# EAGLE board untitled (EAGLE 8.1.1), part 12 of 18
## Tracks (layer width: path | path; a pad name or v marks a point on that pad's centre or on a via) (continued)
S$11975 (continued)
  Bottom 0: 16.56,150.84 16.82,151.06
S$11976
  Bottom 0: 16.82,151.06 17.03,151.35
S$11977
  Bottom 0: 17.03,151.35 17.16,151.67
S$11978
  Bottom 0: 17.16,151.67 17.21,152.02
S$11979
  Bottom 0: 17.21,152.02 17.16,152.36
S$11980
  Bottom 0: 17.16,152.36 17.03,152.69
S$11981
  Bottom 0: 17.03,152.69 16.82,152.97
S$11982
  Bottom 0: 16.82,152.97 16.56,153.2
S$11983
  Bottom 0: 16.56,153.2 16.24,153.35
S$11984
  Bottom 0: 16.24,153.35 15.89,153.41
S$11985
  Bottom 0: 15.89,153.41 15.54,153.39
S$11986
  Bottom 0: 15.54,153.39 15.24,153.29
S$11987
  Bottom 0: 15.24,153.29 16.21,154.26
S$11988
  Bottom 0: 16.21,154.26 16.27,154.33
S$11989
  Bottom 0: 16.27,154.33 16.32,154.41
S$11990
  Bottom 0: 16.32,154.41 16.36,154.49
S$11991
  Bottom 0: 16.36,154.49 16.38,154.57
S$11992
  Bottom 0: 16.38,154.57 16.38,154.66
S$11993
  Bottom 0: 16.38,154.66 16.38,161.85
S$11994
  Bottom 0: 16.38,161.85 16.62,162.02
S$11995
  Bottom 0: 16.62,162.02 16.83,162.28
S$11996
  Bottom 0: 16.83,162.28 16.96,162.57
S$11997
  Bottom 0: 16.96,162.57 17,162.89
S$11998
  Bottom 0: 17,162.89 16.96,163.22
S$11999
  Bottom 0: 16.96,163.22 16.83,163.51
S$12000
  Bottom 0: 16.83,163.51 16.62,163.77
S$12001
  Bottom 0: 16.62,163.77 16.36,163.96
S$12002
  Bottom 0: 16.36,163.96 16.06,164.06
S$12003
  Bottom 0: 16.06,164.06 15.73,164.08
S$12004
  Bottom 0: 15.73,164.08 15.41,164.02
S$12005
  Bottom 0: 15.41,164.02 15.12,163.87
S$12006
  Bottom 0: 15.12,163.87 14.89,163.65
S$12007
  Bottom 0: 14.89,163.65 14.77,163.46
S$12008
  Bottom 0: 14.77,163.46 13.65,163.46
S$12009
  Bottom 0: 13.65,163.46 12.19,164.93
S$12010
  Bottom 0: 12.19,164.93 12.2,164.95
S$12011
  Bottom 0: 12.2,164.95 12.24,165.27
S$12012
  Bottom 0: 12.24,165.27 12.2,165.59
S$12013
  Bottom 0: 12.2,165.59 12.07,165.89
S$12014
  Bottom 0: 12.07,165.89 11.86,166.14
S$12015
  Bottom 0: 11.86,166.14 11.6,166.33
S$12016
  Bottom 0: 11.6,166.33 11.29,166.44
S$12017
  Bottom 0: 11.29,166.44 10.97,166.46
S$12018
  Bottom 0: 10.97,166.46 10.65,166.39
S$12019
  Bottom 0: 10.65,166.39 10.36,166.24
S$12020
  Bottom 0: 10.36,166.24 10.12,166.02
S$12021
  Bottom 0: 10.12,166.02 9.97,165.79
S$12022
  Bottom 0: 9.97,165.79 9.97,170.19
S$12023
  Bottom 0: 9.97,170.19 10.16,169.99
S$12024
  Bottom 0: 10.16,169.99 10.46,169.8
S$12025
  Bottom 0: 10.46,169.8 10.78,169.7
S$12026
  Bottom 0: 10.78,169.7 11.13,169.68
S$12027
  Bottom 0: 11.13,169.68 11.48,169.74
S$12028
  Bottom 0: 11.48,169.74 11.66,169.82
S$12029
  Bottom 0: 11.66,169.82 22,159.49
S$12030
  Bottom 0: 22,159.49 21.9,159.55
S$12031
  Bottom 0: 21.9,159.55 21.61,159.61
S$12032
  Bottom 0: 21.61,159.61 21.3,159.59
S$12033
  Bottom 0: 21.3,159.59 21.02,159.48
S$12034
  Bottom 0: 21.02,159.48 20.78,159.29
S$12035
  Bottom 0: 20.78,159.29 20.61,159.04
S$12036
  Bottom 0: 20.61,159.04 20.52,158.75
S$12037
  Bottom 0: 20.52,158.75 20.52,158.45
S$12038
  Bottom 0: 20.52,158.45 20.61,158.16
S$12039
  Bottom 0: 20.61,158.16 20.78,157.91
S$12040
  Bottom 0: 20.78,157.91 21.02,157.72
S$12041
  Bottom 0: 21.02,157.72 21.3,157.61
S$12042
  Bottom 0: 21.3,157.61 21.61,157.59
S$12043
  Bottom 0: 21.61,157.59 21.9,157.66
S$12044
  Bottom 0: 21.9,157.66 22.16,157.81
S$12045
  Bottom 0: 22.16,157.81 22.29,157.95
S$12046
  Bottom 0: 22.29,157.95 22.29,151.64
S$12047
  Bottom 0: 22.29,151.64 22.16,151.78
S$12048
  Bottom 0: 22.16,151.78 21.9,151.93
S$12049
  Bottom 0: 21.9,151.93 21.61,151.99
S$12050
  Bottom 0: 21.61,151.99 21.3,151.97
S$12051
  Bottom 0: 21.3,151.97 21.02,151.86
S$12052
  Bottom 0: 21.02,151.86 20.78,151.67
S$12053
  Bottom 0: 20.78,151.67 20.61,151.43
S$12054
  Bottom 0: 20.61,151.43 20.52,151.13
S$12055
  Bottom 0: 20.52,151.13 20.52,150.83
S$12056
  Bottom 0: 20.52,150.83 20.61,150.54
S$12057
  Bottom 0: 20.61,150.54 20.78,150.29
S$12058
  Bottom 0: 20.78,150.29 21.02,150.1
S$12059
  Bottom 0: 21.02,150.1 21.3,149.99
S$12060
  Bottom 0: 21.3,149.99 21.61,149.97
S$12061
  Bottom 0: 21.61,149.97 21.9,150.04
S$12062
  Bottom 0: 21.9,150.04 22.16,150.19
S$12063
  Bottom 0: 22.16,150.19 22.29,150.33
S$12064
  Bottom 0: 22.29,150.33 22.29,148.03
S$12065
  Bottom 0: 22.29,148.03 20.8,146.55
S$12066
  Bottom 0: 20.8,146.55 20.76,146.5
S$12067
  Bottom 0: 20.76,146.5 20.72,146.44
S$12068
  Bottom 0: 20.72,146.44 20.69,146.38
S$12069
  Bottom 0: 20.69,146.38 20.67,146.31
S$12070
  Bottom 0: 20.67,146.31 20.67,146.24
S$12071
  Bottom 0: 20.67,146.24 20.67,126.54
S$12072
  Bottom 0: 20.67,126.54 18.82,124.69
S$12073
  Bottom 0: 18.82,124.69 18.78,124.64
S$12074
  Bottom 0: 18.78,124.64 18.74,124.58
S$12075
  Bottom 0: 18.74,124.58 18.71,124.52
S$12076
  Bottom 0: 18.71,124.52 18.69,124.45
S$12077
  Bottom 0: 18.69,124.45 18.69,124.38
S$12078
  Bottom 0: 18.69,124.38 18.69,122.68
S$12079
  Bottom 0: 18.69,122.68 16.99,122.68
S$12080
  Bottom 0: 16.99,122.68 16.91,122.67
S$12081
  Bottom 0: 16.91,122.67 16.84,122.63
S$12082
  Bottom 0: 16.84,122.63 16.78,122.58
S$12083
  Bottom 0: 16.78,122.58 16.74,122.5
S$12084
  Bottom 0: 16.74,122.5 16.73,122.43
S$12085
  Bottom 0: 16.73,122.43 16.73,120.65
S$12086
  Bottom 0: 16.73,120.65 16.74,120.57
S$12087
  Bottom 0: 16.74,120.57 16.78,120.5
S$12088
  Bottom 0: 16.78,120.5 16.84,120.45
S$12089
  Bottom 0: 16.84,120.45 16.91,120.41
S$12090
  Bottom 0: 16.91,120.41 16.99,120.4
S$12091
  Bottom 0: 16.99,120.4 18.77,120.4
S$12092
  Bottom 0: 18.77,120.4 18.84,120.41
S$12093
  Bottom 0: 18.84,120.41 18.91,120.45
S$12094
  Bottom 0: 18.91,120.45 18.92,120.45
S$12095
  Bottom 0: 18.92,120.45 22.51,116.85
S$12096
  Bottom 0: 22.51,116.85 22.51,115.23
S$12097
  Bottom 0: 22.51,115.23 22.36,115.18
S$12098
  Bottom 0: 22.36,115.18 22.07,115
S$12099
  Bottom 0: 22.07,115 21.83,114.74
S$12100
  Bottom 0: 21.83,114.74 21.66,114.43
S$12101
  Bottom 0: 21.66,114.43 21.57,114.09
S$12102
  Bottom 0: 21.57,114.09 21.57,113.75
S$12103
  Bottom 0: 21.57,113.75 21.66,113.41
S$12104
  Bottom 0: 21.66,113.41 21.83,113.1
S$12105
  Bottom 0: 21.83,113.1 22.07,112.84
S$12106
  Bottom 0: 22.07,112.84 22.36,112.65
S$12107
  Bottom 0: 22.36,112.65 22.69,112.55
S$12108
  Bottom 0: 22.69,112.55 23.04,112.53
S$12109
  Bottom 0: 23.04,112.53 23.11,112.54
S$12110
  Bottom 0: 23.11,112.54 13.63,103.06
S$12111
  Bottom 0: 13.63,103.06 11.87,103.06
S$12112
  Bottom 0: 16.69,109.99 17.04,110.05
S$12113
  Bottom 0: 17.04,110.05 17.35,110.2
S$12114
  Bottom 0: 17.35,110.2 17.62,110.42
S$12115
  Bottom 0: 17.62,110.42 17.83,110.71
S$12116
  Bottom 0: 17.83,110.71 17.95,111.03
S$12117
  Bottom 0: 17.95,111.03 18,111.38
S$12118
  Bottom 0: 18,111.38 17.95,111.72
S$12119
  Bottom 0: 17.95,111.72 17.83,112.05
S$12120
  Bottom 0: 17.83,112.05 17.62,112.33
S$12121
  Bottom 0: 17.62,112.33 17.35,112.56
S$12122
  Bottom 0: 17.35,112.56 17.04,112.71
S$12123
  Bottom 0: 17.04,112.71 16.69,112.77
S$12124
  Bottom 0: 16.69,112.77 16.34,112.75
S$12125
  Bottom 0: 16.34,112.75 16.01,112.64
S$12126
  Bottom 0: 16.01,112.64 15.72,112.46
S$12127
  Bottom 0: 15.72,112.46 15.48,112.2
S$12128
  Bottom 0: 15.48,112.2 15.3,111.89
S$12129
  Bottom 0: 15.3,111.89 15.22,111.55
S$12130
  Bottom 0: 15.22,111.55 15.22,111.21
S$12131
  Bottom 0: 15.22,111.21 15.3,110.87
S$12132
  Bottom 0: 15.3,110.87 15.48,110.56
S$12133
  Bottom 0: 15.48,110.56 15.72,110.3
S$12134
  Bottom 0: 15.72,110.3 16.01,110.11
S$12135
  Bottom 0: 16.01,110.11 16.34,110.01
S$12136
  Bottom 0: 16.34,110.01 16.69,109.99
S$12137
  Bottom 0: 19.15,114.17 19.59,114.22
S$12138
  Bottom 0: 19.59,114.22 20.02,114.35
S$12139
  Bottom 0: 20.02,114.35 20.42,114.56
S$12140
  Bottom 0: 20.42,114.56 20.76,114.84
S$12141
  Bottom 0: 20.76,114.84 21.05,115.19
S$12142
  Bottom 0: 21.05,115.19 21.26,115.58
S$12143
  Bottom 0: 21.26,115.58 21.38,116.01
S$12144
  Bottom 0: 21.38,116.01 21.43,116.46
S$12145
  Bottom 0: 21.43,116.46 21.38,116.91
S$12146
  Bottom 0: 21.38,116.91 21.26,117.33
S$12147
  Bottom 0: 21.26,117.33 21.05,117.73
S$12148
  Bottom 0: 21.05,117.73 20.76,118.07
S$12149
  Bottom 0: 20.76,118.07 20.42,118.36
S$12150
  Bottom 0: 20.42,118.36 20.02,118.57
S$12151
  Bottom 0: 20.02,118.57 19.59,118.7
S$12152
  Bottom 0: 19.59,118.7 19.15,118.75
S$12153
  Bottom 0: 19.15,118.75 18.7,118.7
S$12154
  Bottom 0: 18.7,118.7 18.27,118.57
S$12155
  Bottom 0: 18.27,118.57 17.88,118.36
S$12156
  Bottom 0: 17.88,118.36 17.53,118.07
S$12157
  Bottom 0: 17.53,118.07 17.24,117.73
S$12158
  Bottom 0: 17.24,117.73 17.03,117.33
S$12159
  Bottom 0: 17.03,117.33 16.91,116.91
S$12160
  Bottom 0: 16.91,116.91 16.86,116.46
S$12161
  Bottom 0: 16.86,116.46 16.91,116.01
S$12162
  Bottom 0: 16.91,116.01 17.03,115.58
S$12163
  Bottom 0: 17.03,115.58 17.24,115.19
S$12164
  Bottom 0: 17.24,115.19 17.53,114.84
S$12165
  Bottom 0: 17.53,114.84 17.88,114.56
S$12166
  Bottom 0: 17.88,114.56 18.27,114.35
S$12167
  Bottom 0: 18.27,114.35 18.7,114.22
S$12168
  Bottom 0: 18.7,114.22 19.15,114.17
S$12169
  Bottom 0: 297.48,103.13 297.48,103.37
S$12170
  Bottom 0: 297.48,103.37 297.47,103.44
S$12171
  Bottom 0: 297.47,103.44 297.43,103.52
S$12172
  Bottom 0: 297.43,103.52 297.37,103.57
S$12173
  Bottom 0: 297.37,103.57 297.3,103.61
S$12174
  Bottom 0: 297.3,103.61 297.23,103.62
S$12175
  Bottom 0: 297.23,103.62 296.15,103.62
S$12176
  Bottom 0: 296.15,103.62 296.15,103.74
S$12177
  Bottom 0: 296.15,103.74 296.13,103.8
S$12178
  Bottom 0: 296.13,103.8 296.13,103.86
S$12179
  Bottom 0: 296.13,103.86 296.1,103.91
S$12180
  Bottom 0: 296.1,103.91 296.09,103.97
S$12181
  Bottom 0: 296.09,103.97 296.05,104
S$12182
  Bottom 0: 296.05,104 296.02,104.05
S$12183
  Bottom 0: 296.02,104.05 294.98,105.1
S$12184
  Bottom 0: 294.98,105.1 295,105.12
S$12185
  Bottom 0: 295,105.12 295.12,105.42
S$12186
  Bottom 0: 295.12,105.42 295.17,105.74
S$12187
  Bottom 0: 295.17,105.74 295.12,106.06
S$12188
  Bottom 0: 295.12,106.06 295,106.36
S$12189
  Bottom 0: 295,106.36 294.79,106.61
S$12190
  Bottom 0: 294.79,106.61 294.52,106.8
S$12191
  Bottom 0: 294.52,106.8 294.22,106.91
S$12192
  Bottom 0: 294.22,106.91 293.89,106.93
S$12193
  Bottom 0: 293.89,106.93 293.57,106.86
S$12194
  Bottom 0: 293.57,106.86 293.47,106.81
S$12195
  Bottom 0: 293.47,106.81 298.16,111.51
S$12196
  Bottom 0: 298.16,111.51 298.2,111.56
S$12197
  Bottom 0: 298.2,111.56 298.24,111.62
S$12198
  Bottom 0: 298.24,111.62 298.27,111.68
S$12199
  Bottom 0: 298.27,111.68 298.28,111.75
S$12200
  Bottom 0: 298.28,111.75 298.29,111.82
S$12201
  Bottom 0: 298.29,111.82 298.29,112.98
S$12202
  Bottom 0: 298.29,112.98 299.41,114.1
S$12203
  Bottom 0: 299.41,114.1 299.4,114.07
S$12204
  Bottom 0: 299.4,114.07 299.4,113.73
S$12205
  Bottom 0: 299.4,113.73 299.49,113.39
S$12206
  Bottom 0: 299.49,113.39 299.66,113.08
S$12207
  Bottom 0: 299.66,113.08 299.82,112.9
S$12208
  Bottom 0: 299.82,112.9 299.82,103.26
S$12209
  Bottom 0: 299.82,103.26 299.76,103.34
S$12210
  Bottom 0: 299.76,103.34 299.48,103.52
S$12211
  Bottom 0: 299.48,103.52 299.17,103.61
S$12212
  Bottom 0: 299.17,103.61 298.85,103.61
S$12213
  Bottom 0: 298.85,103.61 298.53,103.52
S$12214
  Bottom 0: 298.53,103.52 298.44,103.46
S$12215
  Bottom 0: 298.44,103.46 298.32,103.48
S$12216
  Bottom 0: 298.32,103.48 298.02,103.46
S$12217
  Bottom 0: 298.02,103.46 297.74,103.35
S$12218
  Bottom 0: 297.74,103.35 297.5,103.17
S$12219
  Bottom 0: 297.5,103.17 297.48,103.13
S$12220
  Bottom 0: 300.71,106.53 300.71,112.52
S$12221
  Bottom 0: 300.71,112.52 300.87,112.51
S$12222
  Bottom 0: 300.87,112.51 301.18,112.56
S$12223
  Bottom 0: 301.18,112.56 301.29,112.53
S$12224
  Bottom 0: 301.29,112.53 301.63,112.51
S$12225
  Bottom 0: 301.63,112.51 301.98,112.57
S$12226
  Bottom 0: 301.98,112.57 302.3,112.72
S$12227
  Bottom 0: 302.3,112.72 302.56,112.94
S$12228
  Bottom 0: 302.56,112.94 302.63,113.03
S$12229
  Bottom 0: 302.63,113.03 302.63,107.58
S$12230
  Bottom 0: 302.63,107.58 301.93,106.88
S$12231
  Bottom 0: 301.93,106.88 301.84,106.91
S$12232
  Bottom 0: 301.84,106.91 301.51,106.93
S$12233
  Bottom 0: 301.51,106.93 301.19,106.86
S$12234
  Bottom 0: 301.19,106.86 300.9,106.72
S$12235
  Bottom 0: 300.9,106.72 300.71,106.53
S$12236
  Bottom 0: 34.94,107.82 21.52,121.24
S$12237
  Bottom 0: 21.52,121.24 21.56,121.54
S$12238
  Bottom 0: 21.56,121.54 21.51,121.86
S$12239
  Bottom 0: 21.51,121.86 21.38,122.16
S$12240
  Bottom 0: 21.38,122.16 21.16,122.4
S$12241
  Bottom 0: 21.16,122.4 20.89,122.58
S$12242
  Bottom 0: 20.89,122.58 20.58,122.67
S$12243
  Bottom 0: 20.58,122.67 20.25,122.67
S$12244
  Bottom 0: 20.25,122.67 19.94,122.58
S$12245
  Bottom 0: 19.94,122.58 19.67,122.4
S$12246
  Bottom 0: 19.67,122.4 19.57,122.29
S$12247
  Bottom 0: 19.57,122.29 19.57,124.2
S$12248
  Bottom 0: 19.57,124.2 21.42,126.04
S$12249
  Bottom 0: 21.42,126.04 21.47,126.1
S$12250
  Bottom 0: 21.47,126.1 21.5,126.15
S$12251
  Bottom 0: 21.5,126.15 21.53,126.22
S$12252
  Bottom 0: 21.53,126.22 21.55,126.28
S$12253
  Bottom 0: 21.55,126.28 21.55,126.36
S$12254
  Bottom 0: 21.55,126.36 21.55,146.06
S$12255
  Bottom 0: 21.55,146.06 23.04,147.54
S$12256
  Bottom 0: 23.04,147.54 23.09,147.59
S$12257
  Bottom 0: 23.09,147.59 23.12,147.65
S$12258
  Bottom 0: 23.12,147.65 23.16,147.71
S$12259
  Bottom 0: 23.16,147.71 23.17,147.78
S$12260
  Bottom 0: 23.17,147.78 23.18,147.85
S$12261
  Bottom 0: 23.18,147.85 23.18,152.26
S$12262
  Bottom 0: 23.18,152.26 29.48,152.26
S$12263
  Bottom 0: 29.48,152.26 29.58,152.15
S$12264
  Bottom 0: 29.58,152.15 29.8,152.04
S$12265
  Bottom 0: 29.8,152.04 30.05,152.02
S$12266
  Bottom 0: 30.05,152.02 30.3,152.09
S$12267
  Bottom 0: 30.3,152.09 30.39,152.16
S$12268
  Bottom 0: 30.39,152.16 30.47,152.06
S$12269
  Bottom 0: 30.47,152.06 30.67,151.85
S$12270
  Bottom 0: 30.67,151.85 30.72,151.81
S$12271
  Bottom 0: 30.72,151.81 30.78,151.77
S$12272
  Bottom 0: 30.78,151.77 30.85,151.74
S$12273
  Bottom 0: 30.85,151.74 30.91,151.72
S$12274
  Bottom 0: 30.91,151.72 30.98,151.72
S$12275
  Bottom 0: 30.98,151.72 32.56,151.72
S$12276
  Bottom 0: 32.56,151.72 33.42,150.86
S$12277
  Bottom 0: 33.42,150.86 33.36,150.87
S$12278
  Bottom 0: 33.36,150.87 33.01,150.85
S$12279
  Bottom 0: 33.01,150.85 32.68,150.74
S$12280
  Bottom 0: 32.68,150.74 32.65,150.73
S$12281
  Bottom 0: 32.65,150.73 32.08,151.3
S$12282
  Bottom 0: 32.08,151.3 32.02,151.34
S$12283
  Bottom 0: 32.02,151.34 31.96,151.38
S$12284
  Bottom 0: 31.96,151.38 31.9,151.41
S$12285
  Bottom 0: 31.9,151.41 31.83,151.43
S$12286
  Bottom 0: 31.83,151.43 31.77,151.43
S$12287
  Bottom 0: 31.77,151.43 27.19,151.43
S$12288
  Bottom 0: 27.19,151.43 27.13,151.56
S$12289
  Bottom 0: 27.13,151.56 26.92,151.78
S$12290
  Bottom 0: 26.92,151.78 26.66,151.93
S$12291
  Bottom 0: 26.66,151.93 26.36,152
S$12292
  Bottom 0: 26.36,152 26.06,151.98
S$12293
  Bottom 0: 26.06,151.98 25.78,151.87
S$12294
  Bottom 0: 25.78,151.87 25.54,151.68
S$12295
  Bottom 0: 25.54,151.68 25.37,151.43
S$12296
  Bottom 0: 25.37,151.43 25.28,151.14
S$12297
  Bottom 0: 25.28,151.14 25.28,150.84
S$12298
  Bottom 0: 25.28,150.84 25.37,150.55
S$12299
  Bottom 0: 25.37,150.55 25.54,150.3
S$12300
  Bottom 0: 25.54,150.3 25.78,150.11
S$12301
  Bottom 0: 25.78,150.11 26.06,150
S$12302
  Bottom 0: 26.06,150 26.36,149.98
S$12303
  Bottom 0: 26.36,149.98 26.66,150.04
S$12304
  Bottom 0: 26.66,150.04 26.92,150.19
S$12305
  Bottom 0: 26.92,150.19 27.13,150.41
S$12306
  Bottom 0: 27.13,150.41 27.19,150.55
S$12307
  Bottom 0: 27.19,150.55 31.58,150.55
S$12308
  Bottom 0: 31.58,150.55 32.03,150.09
S$12309
  Bottom 0: 32.03,150.09 31.97,149.99
S$12310
  Bottom 0: 31.97,149.99 31.89,149.65
S$12311
  Bottom 0: 31.89,149.65 31.89,149.3
S$12312
  Bottom 0: 31.89,149.3 31.97,148.97
S$12313
  Bottom 0: 31.97,148.97 32.15,148.66
S$12314
  Bottom 0: 32.15,148.66 32.38,148.4
S$12315
  Bottom 0: 32.38,148.4 32.68,148.21
S$12316
  Bottom 0: 32.68,148.21 33.01,148.11
S$12317
  Bottom 0: 33.01,148.11 33.36,148.09
S$12318
  Bottom 0: 33.36,148.09 33.7,148.15
S$12319
  Bottom 0: 33.7,148.15 34.02,148.3
S$12320
  Bottom 0: 34.02,148.3 34.29,148.52
S$12321
  Bottom 0: 34.29,148.52 34.5,148.81
S$12322
  Bottom 0: 34.5,148.81 34.62,149.13
S$12323
  Bottom 0: 34.62,149.13 34.67,149.48
S$12324
  Bottom 0: 34.67,149.48 34.65,149.63
S$12325
  Bottom 0: 34.65,149.63 40.24,144.04
S$12326
  Bottom 0: 40.24,144.04 40.22,144.02
S$12327
  Bottom 0: 40.22,144.02 40.19,143.96
S$12328
  Bottom 0: 40.19,143.96 40.16,143.89
S$12329
  Bottom 0: 40.16,143.89 40.14,143.82
S$12330
  Bottom 0: 40.14,143.82 40.13,143.75
S$12331
  Bottom 0: 40.13,143.75 40.13,141.73
S$12332
  Bottom 0: 40.13,141.73 39.75,141.73
S$12333
  Bottom 0: 39.75,141.73 39.75,141.86
S$12334
  Bottom 0: 39.75,141.86 39.69,142.08
S$12335
  Bottom 0: 39.69,142.08 39.52,142.24
S$12336
  Bottom 0: 39.52,142.24 39.3,142.3
S$12337
  Bottom 0: 39.3,142.3 38.94,142.3
S$12338
  Bottom 0: 38.94,142.3 37.85,143.39
S$12339
  Bottom 0: 37.85,143.39 37.91,143.52
S$12340
  Bottom 0: 37.91,143.52 37.96,143.84
S$12341
  Bottom 0: 37.96,143.84 37.91,144.16
S$12342
  Bottom 0: 37.91,144.16 37.79,144.47
S$12343
  Bottom 0: 37.79,144.47 37.58,144.72
S$12344
  Bottom 0: 37.58,144.72 37.31,144.91
S$12345
  Bottom 0: 37.31,144.91 37.01,145.01
S$12346
  Bottom 0: 37.01,145.01 36.69,145.03
S$12347
  Bottom 0: 36.69,145.03 36.37,144.97
S$12348
  Bottom 0: 36.37,144.97 36.08,144.82
S$12349
  Bottom 0: 36.08,144.82 35.84,144.6
S$12350
  Bottom 0: 35.84,144.6 35.67,144.32
S$12351
  Bottom 0: 35.67,144.32 35.59,144.01
S$12352
  Bottom 0: 35.59,144.01 35.59,143.68
S$12353
  Bottom 0: 35.59,143.68 35.67,143.37
S$12354
  Bottom 0: 35.67,143.37 35.84,143.09
S$12355
  Bottom 0: 35.84,143.09 36.08,142.87
S$12356
  Bottom 0: 36.08,142.87 36.37,142.72
S$12357
  Bottom 0: 36.37,142.72 36.69,142.66
S$12358
  Bottom 0: 36.69,142.66 37.01,142.68
S$12359
  Bottom 0: 37.01,142.68 37.23,142.75
S$12360
  Bottom 0: 37.23,142.75 38.29,141.7
S$12361
  Bottom 0: 38.29,141.7 38.27,141.68
S$12362
  Bottom 0: 38.27,141.68 38.21,141.62
S$12363
  Bottom 0: 38.21,141.62 38.17,141.55
S$12364
  Bottom 0: 38.17,141.55 38.16,141.48
S$12365
  Bottom 0: 38.16,141.48 38.16,139.7
S$12366
  Bottom 0: 38.16,139.7 38.17,139.62
S$12367
  Bottom 0: 38.17,139.62 38.21,139.55
S$12368
  Bottom 0: 38.21,139.55 38.27,139.5
S$12369
  Bottom 0: 38.27,139.5 38.34,139.46
S$12370
  Bottom 0: 38.34,139.46 38.41,139.45
S$12371
  Bottom 0: 38.41,139.45 40.13,139.45
S$12372
  Bottom 0: 40.13,139.45 40.13,139.14
S$12373
  Bottom 0: 40.13,139.14 36.2,135.2
S$12374
  Bottom 0: 36.2,135.2 36.16,135.15
S$12375
  Bottom 0: 36.16,135.15 36.12,135.09
S$12376
  Bottom 0: 36.12,135.09 36.1,135.03
S$12377
  Bottom 0: 36.1,135.03 36.08,134.97
S$12378
  Bottom 0: 36.08,134.97 36.08,134.89
S$12379
  Bottom 0: 36.08,134.89 36.08,129.7
S$12380
  Bottom 0: 36.08,129.7 36.08,129.63
S$12381
  Bottom 0: 36.08,129.63 36.1,129.56
S$12382
  Bottom 0: 36.1,129.56 36.12,129.5
S$12383
  Bottom 0: 36.12,129.5 36.16,129.44
S$12384
  Bottom 0: 36.16,129.44 36.2,129.39
S$12385
  Bottom 0: 36.2,129.39 46.11,119.48
S$12386
  Bottom 0: 46.11,119.48 46.17,119.44
S$12387
  Bottom 0: 46.17,119.44 46.23,119.39
S$12388
  Bottom 0: 46.23,119.39 46.29,119.37
S$12389
  Bottom 0: 46.29,119.37 46.36,119.36
S$12390
  Bottom 0: 46.36,119.36 46.43,119.35
S$12391
  Bottom 0: 46.43,119.35 49.98,119.35
S$12392
  Bottom 0: 49.98,119.35 50.68,118.66
S$12393
  Bottom 0: 50.68,118.66 50.55,118.7
S$12394
  Bottom 0: 50.55,118.7 50.1,118.75
S$12395
  Bottom 0: 50.1,118.75 49.65,118.7
S$12396
  Bottom 0: 49.65,118.7 49.22,118.57
S$12397
  Bottom 0: 49.22,118.57 48.83,118.36
S$12398
  Bottom 0: 48.83,118.36 48.48,118.07
S$12399
  Bottom 0: 48.48,118.07 48.2,117.73
S$12400
  Bottom 0: 48.2,117.73 47.98,117.33
S$12401
  Bottom 0: 47.98,117.33 47.86,116.91
S$12402
  Bottom 0: 47.86,116.91 47.81,116.46
S$12403
  Bottom 0: 47.81,116.46 47.86,116.01
S$12404
  Bottom 0: 47.86,116.01 47.98,115.58
S$12405
  Bottom 0: 47.98,115.58 48.2,115.19
S$12406
  Bottom 0: 48.2,115.19 48.48,114.84
S$12407
  Bottom 0: 48.48,114.84 48.83,114.56
S$12408
  Bottom 0: 48.83,114.56 49.22,114.35
S$12409
  Bottom 0: 49.22,114.35 49.65,114.22
S$12410
  Bottom 0: 49.65,114.22 50.1,114.17
S$12411
  Bottom 0: 50.1,114.17 50.55,114.22
S$12412
  Bottom 0: 50.55,114.22 50.97,114.35
S$12413
  Bottom 0: 50.97,114.35 51.37,114.56
S$12414
  Bottom 0: 51.37,114.56 51.71,114.84
S$12415
  Bottom 0: 51.71,114.84 52,115.19
S$12416
  Bottom 0: 52,115.19 52.21,115.58
S$12417
  Bottom 0: 52.21,115.58 52.34,116.01
S$12418
  Bottom 0: 52.34,116.01 52.38,116.46
S$12419
  Bottom 0: 52.38,116.46 52.34,116.91
S$12420
  Bottom 0: 52.34,116.91 52.3,117.04
S$12421
  Bottom 0: 52.3,117.04 53.47,115.87
S$12422
  Bottom 0: 53.47,115.87 53.47,115.23
S$12423
  Bottom 0: 53.47,115.23 53.31,115.18
S$12424
  Bottom 0: 53.31,115.18 53.02,115
S$12425
  Bottom 0: 53.02,115 52.78,114.74
S$12426
  Bottom 0: 52.78,114.74 52.61,114.43
S$12427
  Bottom 0: 52.61,114.43 52.52,114.09
S$12428
  Bottom 0: 52.52,114.09 52.52,113.75
S$12429
  Bottom 0: 52.52,113.75 52.61,113.41
S$12430
  Bottom 0: 52.61,113.41 52.78,113.1
S$12431
  Bottom 0: 52.78,113.1 53.02,112.84
S$12432
  Bottom 0: 53.02,112.84 53.31,112.65
S$12433
  Bottom 0: 53.31,112.65 53.65,112.55
S$12434
  Bottom 0: 53.65,112.55 53.99,112.53
S$12435
  Bottom 0: 53.99,112.53 54.34,112.59
S$12436
  Bottom 0: 54.34,112.59 54.65,112.74
S$12437
  Bottom 0: 54.65,112.74 54.92,112.96
S$12438
  Bottom 0: 54.92,112.96 55.11,113.21
S$12439
  Bottom 0: 55.11,113.21 55.11,107.82
S$12440
  Bottom 0: 55.11,107.82 34.94,107.82
S$12441
  Bottom 0: 47.65,109.99 47.99,110.05
S$12442
  Bottom 0: 47.99,110.05 48.3,110.2
S$12443
  Bottom 0: 48.3,110.2 48.58,110.42
S$12444
  Bottom 0: 48.58,110.42 48.78,110.71
S$12445
  Bottom 0: 48.78,110.71 48.91,111.03
S$12446
  Bottom 0: 48.91,111.03 48.96,111.38
S$12447
  Bottom 0: 48.96,111.38 48.91,111.72
S$12448
  Bottom 0: 48.91,111.72 48.78,112.05
S$12449
  Bottom 0: 48.78,112.05 48.58,112.33
S$12450
  Bottom 0: 48.58,112.33 48.3,112.56
S$12451
  Bottom 0: 48.3,112.56 47.99,112.71
S$12452
  Bottom 0: 47.99,112.71 47.65,112.77
S$12453
  Bottom 0: 47.65,112.77 47.3,112.75
S$12454
  Bottom 0: 47.3,112.75 46.96,112.64
S$12455
  Bottom 0: 46.96,112.64 46.94,112.63
S$12456
  Bottom 0: 46.94,112.63 46.38,113.19
S$12457
  Bottom 0: 46.38,113.19 46.32,113.24
S$12458
  Bottom 0: 46.32,113.24 46.26,113.27
S$12459
  Bottom 0: 46.26,113.27 46.2,113.3
S$12460
  Bottom 0: 46.2,113.3 46.13,113.32
S$12461
  Bottom 0: 46.13,113.32 46.06,113.33
S$12462
  Bottom 0: 46.06,113.33 42.68,113.33
S$12463
  Bottom 0: 42.68,113.33 42.61,113.46
S$12464
  Bottom 0: 42.61,113.46 42.41,113.67
S$12465
  Bottom 0: 42.41,113.67 42.14,113.83
S$12466
  Bottom 0: 42.14,113.83 41.85,113.89
S$12467
  Bottom 0: 41.85,113.89 41.54,113.87
S$12468
  Bottom 0: 41.54,113.87 41.27,113.76
S$12469
  Bottom 0: 41.27,113.76 41.02,113.57
S$12470
  Bottom 0: 41.02,113.57 40.86,113.33
S$12471
  Bottom 0: 40.86,113.33 40.77,113.03
S$12472
  Bottom 0: 40.77,113.03 40.77,112.73
S$12473
  Bottom 0: 40.77,112.73 40.86,112.44
S$12474
  Bottom 0: 40.86,112.44 41.02,112.19
S$12475
  Bottom 0: 41.02,112.19 41.27,112
S$12476
  Bottom 0: 41.27,112 41.54,111.89
S$12477
  Bottom 0: 41.54,111.89 41.85,111.87
S$12478
  Bottom 0: 41.85,111.87 42.14,111.94
S$12479
  Bottom 0: 42.14,111.94 42.41,112.09
S$12480
  Bottom 0: 42.41,112.09 42.61,112.31
S$12481
  Bottom 0: 42.61,112.31 42.68,112.44
S$12482
  Bottom 0: 42.68,112.44 45.88,112.44
S$12483
  Bottom 0: 45.88,112.44 46.32,112
S$12484
  Bottom 0: 46.32,112 46.26,111.89
S$12485
  Bottom 0: 46.26,111.89 46.17,111.55
S$12486
  Bottom 0: 46.17,111.55 46.17,111.21
S$12487
  Bottom 0: 46.17,111.21 46.26,110.87
S$12488
  Bottom 0: 46.26,110.87 46.43,110.56
S$12489
  Bottom 0: 46.43,110.56 46.67,110.3
S$12490
  Bottom 0: 46.67,110.3 46.96,110.11
S$12491
  Bottom 0: 46.96,110.11 47.3,110.01
S$12492
  Bottom 0: 47.3,110.01 47.65,109.99
S$12493
  Bottom 0: 39.47,111.88 39.76,111.94
S$12494
  Bottom 0: 39.76,111.94 40.02,112.09
S$12495
  Bottom 0: 40.02,112.09 40.23,112.31
S$12496
  Bottom 0: 40.23,112.31 40.36,112.59
S$12497
  Bottom 0: 40.36,112.59 40.41,112.89
S$12498
  Bottom 0: 40.41,112.89 40.36,113.19
S$12499
  Bottom 0: 40.36,113.19 40.23,113.46
S$12500
  Bottom 0: 40.23,113.46 40.02,113.68
S$12501
  Bottom 0: 40.02,113.68 39.76,113.83
S$12502
  Bottom 0: 39.76,113.83 39.47,113.9
S$12503
  Bottom 0: 39.47,113.9 39.16,113.88
S$12504
  Bottom 0: 39.16,113.88 38.88,113.77
S$12505
  Bottom 0: 38.88,113.77 38.64,113.58
S$12506
  Bottom 0: 38.64,113.58 38.48,113.33
S$12507
  Bottom 0: 38.48,113.33 38.38,113.04
S$12508
  Bottom 0: 38.38,113.04 38.38,112.73
S$12509
  Bottom 0: 38.38,112.73 38.48,112.45
S$12510
  Bottom 0: 38.48,112.45 38.64,112.2
S$12511
  Bottom 0: 38.64,112.2 38.88,112.01
S$12512
  Bottom 0: 38.88,112.01 39.16,111.9
S$12513
  Bottom 0: 39.16,111.9 39.47,111.88
S$12514
  Bottom 0: 41.85,119.49 42.14,119.56
S$12515
  Bottom 0: 42.14,119.56 42.41,119.71
S$12516
  Bottom 0: 42.41,119.71 42.61,119.93
S$12517
  Bottom 0: 42.61,119.93 42.74,120.2
S$12518
  Bottom 0: 42.74,120.2 42.79,120.5
S$12519
  Bottom 0: 42.79,120.5 42.74,120.8
S$12520
  Bottom 0: 42.74,120.8 42.61,121.08
S$12521
  Bottom 0: 42.61,121.08 42.41,121.3
S$12522
  Bottom 0: 42.41,121.3 42.14,121.45
S$12523
  Bottom 0: 42.14,121.45 41.85,121.51
S$12524
  Bottom 0: 41.85,121.51 41.54,121.49
S$12525
  Bottom 0: 41.54,121.49 41.27,121.38
S$12526
  Bottom 0: 41.27,121.38 41.02,121.19
S$12527
  Bottom 0: 41.02,121.19 40.86,120.94
S$12528
  Bottom 0: 40.86,120.94 40.77,120.66
S$12529
  Bottom 0: 40.77,120.66 40.77,120.35
S$12530
  Bottom 0: 40.77,120.35 40.86,120.06
S$12531
  Bottom 0: 40.86,120.06 41.02,119.81
S$12532
  Bottom 0: 41.02,119.81 41.27,119.62
S$12533
  Bottom 0: 41.27,119.62 41.54,119.51
S$12534
  Bottom 0: 41.54,119.51 41.85,119.49
S$12535
  Bottom 0: 39.47,119.5 39.76,119.56
S$12536
  Bottom 0: 39.76,119.56 40.02,119.72
S$12537
  Bottom 0: 40.02,119.72 40.23,119.93
S$12538
  Bottom 0: 40.23,119.93 40.36,120.21
S$12539
  Bottom 0: 40.36,120.21 40.41,120.51
S$12540
  Bottom 0: 40.41,120.51 40.36,120.81
S$12541
  Bottom 0: 40.36,120.81 40.23,121.08
S$12542
  Bottom 0: 40.23,121.08 40.02,121.3
S$12543
  Bottom 0: 40.02,121.3 39.76,121.45
S$12544
  Bottom 0: 39.76,121.45 39.47,121.52
S$12545
  Bottom 0: 39.47,121.52 39.16,121.5
S$12546
  Bottom 0: 39.16,121.5 38.88,121.39
S$12547
  Bottom 0: 38.88,121.39 38.64,121.2
S$12548
  Bottom 0: 38.64,121.2 38.48,120.95
S$12549
  Bottom 0: 38.48,120.95 38.38,120.66
S$12550
  Bottom 0: 38.38,120.66 38.38,120.36
S$12551
  Bottom 0: 38.38,120.36 38.48,120.07
S$12552
  Bottom 0: 38.48,120.07 38.64,119.82
S$12553
  Bottom 0: 38.64,119.82 38.88,119.63
S$12554
  Bottom 0: 38.88,119.63 39.16,119.52
S$12555
  Bottom 0: 39.16,119.52 39.47,119.5
S$12556
  Bottom 0: 32.32,124.97 32.62,125.03
S$12557
  Bottom 0: 32.62,125.03 32.88,125.19
S$12558
  Bottom 0: 32.88,125.19 33.09,125.41
S$12559
  Bottom 0: 33.09,125.41 33.22,125.68
S$12560
  Bottom 0: 33.22,125.68 33.26,125.98
S$12561
  Bottom 0: 33.26,125.98 33.22,126.28
S$12562
  Bottom 0: 33.22,126.28 33.09,126.55
S$12563
  Bottom 0: 33.09,126.55 32.88,126.77
S$12564
  Bottom 0: 32.88,126.77 32.62,126.92
S$12565
  Bottom 0: 32.62,126.92 32.32,126.99
S$12566
  Bottom 0: 32.32,126.99 32.02,126.97
S$12567
  Bottom 0: 32.02,126.97 31.74,126.86
S$12568
  Bottom 0: 31.74,126.86 31.5,126.67
S$12569
  Bottom 0: 31.5,126.67 31.33,126.42
S$12570
  Bottom 0: 31.33,126.42 31.24,126.13
S$12571
  Bottom 0: 31.24,126.13 31.24,125.83
S$12572
  Bottom 0: 31.24,125.83 31.33,125.54
S$12573
  Bottom 0: 31.33,125.54 31.5,125.29
S$12574
  Bottom 0: 31.5,125.29 31.74,125.1
S$12575
  Bottom 0: 31.74,125.1 32.02,124.99
S$12576
  Bottom 0: 32.02,124.99 32.32,124.97
S$12577
  Bottom 0: 22.79,124.97 23.09,125.03
S$12578
  Bottom 0: 23.09,125.03 23.35,125.19
S$12579
  Bottom 0: 23.35,125.19 23.56,125.41
S$12580
  Bottom 0: 23.56,125.41 23.69,125.68
S$12581
  Bottom 0: 23.69,125.68 23.73,125.98
S$12582
  Bottom 0: 23.73,125.98 23.69,126.28
S$12583
  Bottom 0: 23.69,126.28 23.56,126.55
S$12584
  Bottom 0: 23.56,126.55 23.35,126.77
S$12585
  Bottom 0: 23.35,126.77 23.09,126.92
S$12586
  Bottom 0: 23.09,126.92 22.79,126.99
S$12587
  Bottom 0: 22.79,126.99 22.49,126.97
S$12588
  Bottom 0: 22.49,126.97 22.21,126.86
S$12589
  Bottom 0: 22.21,126.86 21.97,126.67
S$12590
  Bottom 0: 21.97,126.67 21.8,126.42
S$12591
  Bottom 0: 21.8,126.42 21.71,126.13
S$12592
  Bottom 0: 21.71,126.13 21.71,125.83
S$12593
  Bottom 0: 21.71,125.83 21.8,125.54
S$12594
  Bottom 0: 21.8,125.54 21.97,125.29
S$12595
  Bottom 0: 21.97,125.29 22.21,125.1
S$12596
  Bottom 0: 22.21,125.1 22.49,124.99
S$12597
  Bottom 0: 22.49,124.99 22.79,124.97
S$12598
  Bottom 0: 32.32,132.59 32.62,132.65
S$12599
  Bottom 0: 32.62,132.65 32.88,132.81
S$12600
  Bottom 0: 32.88,132.81 33.09,133.03
S$12601
  Bottom 0: 33.09,133.03 33.22,133.3
S$12602
  Bottom 0: 33.22,133.3 33.26,133.6
S$12603
  Bottom 0: 33.26,133.6 33.22,133.9
S$12604
  Bottom 0: 33.22,133.9 33.09,134.17
S$12605
  Bottom 0: 33.09,134.17 32.88,134.39
S$12606
  Bottom 0: 32.88,134.39 32.62,134.54
S$12607
  Bottom 0: 32.62,134.54 32.32,134.61
S$12608
  Bottom 0: 32.32,134.61 32.02,134.59
S$12609
  Bottom 0: 32.02,134.59 31.74,134.48
S$12610
  Bottom 0: 31.74,134.48 31.5,134.29
S$12611
  Bottom 0: 31.5,134.29 31.33,134.04
S$12612
  Bottom 0: 31.33,134.04 31.24,133.75
S$12613
  Bottom 0: 31.24,133.75 31.24,133.45
S$12614
  Bottom 0: 31.24,133.45 31.33,133.16
S$12615
  Bottom 0: 31.33,133.16 31.5,132.91
S$12616
  Bottom 0: 31.5,132.91 31.74,132.72
S$12617
  Bottom 0: 31.74,132.72 32.02,132.61
S$12618
  Bottom 0: 32.02,132.61 32.32,132.59
S$12619
  Bottom 0: 22.79,132.59 23.09,132.65
S$12620
  Bottom 0: 23.09,132.65 23.35,132.81
S$12621
  Bottom 0: 23.35,132.81 23.56,133.03
S$12622
  Bottom 0: 23.56,133.03 23.69,133.3
S$12623
  Bottom 0: 23.69,133.3 23.73,133.6
S$12624
  Bottom 0: 23.73,133.6 23.69,133.9
S$12625
  Bottom 0: 23.69,133.9 23.56,134.17
S$12626
  Bottom 0: 23.56,134.17 23.35,134.39
S$12627
  Bottom 0: 23.35,134.39 23.09,134.54
S$12628
  Bottom 0: 23.09,134.54 22.79,134.61
S$12629
  Bottom 0: 22.79,134.61 22.49,134.59
S$12630
  Bottom 0: 22.49,134.59 22.21,134.48
S$12631
  Bottom 0: 22.21,134.48 21.97,134.29
S$12632
  Bottom 0: 21.97,134.29 21.8,134.04
S$12633
  Bottom 0: 21.8,134.04 21.71,133.75
S$12634
  Bottom 0: 21.71,133.75 21.71,133.45
S$12635
  Bottom 0: 21.71,133.45 21.8,133.16
S$12636
  Bottom 0: 21.8,133.16 21.97,132.91
S$12637
  Bottom 0: 21.97,132.91 22.21,132.72
S$12638
  Bottom 0: 22.21,132.72 22.49,132.61
S$12639
  Bottom 0: 22.49,132.61 22.79,132.59
S$12640
  Bottom 0: 29.01,133.44 29.36,133.65
S$12641
  Bottom 0: 29.36,133.65 29.77,133.98
S$12642
  Bottom 0: 29.77,133.98 30.13,134.38
S$12643
  Bottom 0: 30.13,134.38 30.41,134.83
S$12644
  Bottom 0: 30.41,134.83 30.42,134.84
S$12645
  Bottom 0: 30.42,134.84 29.01,134.84
S$12646
  Bottom 0: 29.01,134.84 29.01,133.44
S$12647
  Bottom 0: 25.96,133.44 25.96,134.84
S$12648
  Bottom 0: 25.96,134.84 24.57,134.84
S$12649
  Bottom 0: 24.57,134.84 24.7,134.6
S$12650
  Bottom 0: 24.7,134.6 25.01,134.17
S$12651
  Bottom 0: 25.01,134.17 25.4,133.81
S$12652
  Bottom 0: 25.4,133.81 25.84,133.5
S$12653
  Bottom 0: 25.84,133.5 25.96,133.44
S$12654
  Bottom 0: 29.01,137.89 30.42,137.89
S$12655
  Bottom 0: 30.42,137.89 30.41,137.9
S$12656
  Bottom 0: 30.41,137.9 30.13,138.34
S$12657
  Bottom 0: 30.13,138.34 29.77,138.75
S$12658
  Bottom 0: 29.77,138.75 29.36,139.08
S$12659
  Bottom 0: 29.36,139.08 29.01,139.28
S$12660
  Bottom 0: 29.01,139.28 29.01,137.89
S$12661
  Bottom 0: 24.57,137.89 25.96,137.89
S$12662
  Bottom 0: 25.96,137.89 25.96,139.28
S$12663
  Bottom 0: 25.96,139.28 25.84,139.22
S$12664
  Bottom 0: 25.84,139.22 25.4,138.92
S$12665
  Bottom 0: 25.4,138.92 25.01,138.55
S$12666
  Bottom 0: 25.01,138.55 24.7,138.12
S$12667
  Bottom 0: 24.7,138.12 24.57,137.89
S$12668
  Bottom 0: 147.97,110.19 147.97,113.2
S$12669
  Bottom 0: 147.97,113.2 148.03,113.1
S$12670
  Bottom 0: 148.03,113.1 148.27,112.84
S$12671
  Bottom 0: 148.27,112.84 148.56,112.65
S$12672
  Bottom 0: 148.56,112.65 148.9,112.55
S$12673
  Bottom 0: 148.9,112.55 149.25,112.53
S$12674
  Bottom 0: 149.25,112.53 149.59,112.59
S$12675
  Bottom 0: 149.59,112.59 149.9,112.74
S$12676
  Bottom 0: 149.9,112.74 150.18,112.96
S$12677
  Bottom 0: 150.18,112.96 150.38,113.25
S$12678
  Bottom 0: 150.38,113.25 150.51,113.57
S$12679
  Bottom 0: 150.51,113.57 150.56,113.92
S$12680
  Bottom 0: 150.56,113.92 150.51,114.26
S$12681
  Bottom 0: 150.51,114.26 150.38,114.59
S$12682
  Bottom 0: 150.38,114.59 150.18,114.87
S$12683
  Bottom 0: 150.18,114.87 149.9,115.1
S$12684
  Bottom 0: 149.9,115.1 149.6,115.25
S$12685
  Bottom 0: 149.6,115.25 149.6,122.89
S$12686
  Bottom 0: 149.6,122.89 149.6,122.96
S$12687
  Bottom 0: 149.6,122.96 149.58,123.02
S$12688
  Bottom 0: 149.58,123.02 149.55,123.09
S$12689
  Bottom 0: 149.55,123.09 149.51,123.14
S$12690
  Bottom 0: 149.51,123.14 149.47,123.2
S$12691
  Bottom 0: 149.47,123.2 149.06,123.61
S$12692
  Bottom 0: 149.06,123.61 149.09,123.6
S$12693
  Bottom 0: 149.09,123.6 149.42,123.62
S$12694
  Bottom 0: 149.42,123.62 149.72,123.73
S$12695
  Bottom 0: 149.72,123.73 149.99,123.92
S$12696
  Bottom 0: 149.99,123.92 150.19,124.17
S$12697
  Bottom 0: 150.19,124.17 150.22,124.22
S$12698
  Bottom 0: 150.22,124.22 152.96,124.22
S$12699
  Bottom 0: 152.96,124.22 153.05,124.23
S$12700
  Bottom 0: 153.05,124.23 153.14,124.25
S$12701
  Bottom 0: 153.14,124.25 153.22,124.28
S$12702
  Bottom 0: 153.22,124.28 153.29,124.33
S$12703
  Bottom 0: 153.29,124.33 153.36,124.39
S$12704
  Bottom 0: 153.36,124.39 160.45,131.48
S$12705
  Bottom 0: 160.45,131.48 167.05,124.88
S$12706
  Bottom 0: 167.05,124.88 167.05,124.63
S$12707
  Bottom 0: 167.05,124.63 167.13,124.31
S$12708
  Bottom 0: 167.13,124.31 167.31,124.04
S$12709
  Bottom 0: 167.31,124.04 167.54,123.81
S$12710
  Bottom 0: 167.54,123.81 167.83,123.67
S$12711
  Bottom 0: 167.83,123.67 168.15,123.6
S$12712
  Bottom 0: 168.15,123.6 168.47,123.62
S$12713
  Bottom 0: 168.47,123.62 168.56,123.65
S$12714
  Bottom 0: 168.56,123.65 169.69,122.53
S$12715
  Bottom 0: 169.69,122.53 169.76,122.46
S$12716
  Bottom 0: 169.76,122.46 169.84,122.42
S$12717
  Bottom 0: 169.84,122.42 169.92,122.38
S$12718
  Bottom 0: 169.92,122.38 170,122.36
S$12719
  Bottom 0: 170,122.36 170.09,122.36
S$12720
  Bottom 0: 170.09,122.36 177.09,122.36
S$12721
  Bottom 0: 177.09,122.36 177.09,121.2
S$12722
  Bottom 0: 177.09,121.2 176.95,121.31
S$12723
  Bottom 0: 176.95,121.31 176.7,121.37
S$12724
  Bottom 0: 176.7,121.37 176.45,121.35
S$12725
  Bottom 0: 176.45,121.35 176.23,121.24
S$12726
  Bottom 0: 176.23,121.24 176.06,121.05
S$12727
  Bottom 0: 176.06,121.05 175.97,120.82
S$12728
  Bottom 0: 175.97,120.82 172.95,117.8
S$12729
  Bottom 0: 172.95,117.8 170.21,117.8
S$12730
  Bottom 0: 170.21,117.8 166.77,121.24
S$12731
  Bottom 0: 166.77,121.24 166.81,121.54
S$12732
  Bottom 0: 166.81,121.54 166.78,121.75
S$12733
  Bottom 0: 166.78,121.75 168.35,120.19
S$12734
  Bottom 0: 168.35,120.19 168.4,120.15
S$12735
  Bottom 0: 168.4,120.15 168.46,120.11
S$12736
  Bottom 0: 168.46,120.11 168.52,120.08
S$12737
  Bottom 0: 168.52,120.08 168.59,120.07
S$12738
  Bottom 0: 168.59,120.07 168.66,120.06
S$12739
  Bottom 0: 168.66,120.06 173.03,120.06
S$12740
  Bottom 0: 173.03,120.06 173.19,119.81
S$12741
  Bottom 0: 173.19,119.81 173.43,119.62
S$12742
  Bottom 0: 173.43,119.62 173.71,119.51
S$12743
  Bottom 0: 173.71,119.51 174.01,119.49
S$12744
  Bottom 0: 174.01,119.49 174.31,119.56
S$12745
  Bottom 0: 174.31,119.56 174.57,119.71
S$12746
  Bottom 0: 174.57,119.71 174.78,119.93
S$12747
  Bottom 0: 174.78,119.93 174.91,120.2
S$12748
  Bottom 0: 174.91,120.2 174.96,120.5
S$12749
  Bottom 0: 174.96,120.5 174.91,120.8
S$12750
  Bottom 0: 174.91,120.8 174.78,121.08
S$12751
  Bottom 0: 174.78,121.08 174.57,121.3
S$12752
  Bottom 0: 174.57,121.3 174.31,121.45
S$12753
  Bottom 0: 174.31,121.45 174.01,121.51
S$12754
  Bottom 0: 174.01,121.51 173.71,121.49
S$12755
  Bottom 0: 173.71,121.49 173.43,121.38
S$12756
  Bottom 0: 173.43,121.38 173.19,121.19
S$12757
  Bottom 0: 173.19,121.19 173.03,120.94
S$12758
  Bottom 0: 173.03,120.94 168.85,120.94
S$12759
  Bottom 0: 168.85,120.94 166.67,123.12
S$12760
  Bottom 0: 166.67,123.12 166.61,123.17
S$12761
  Bottom 0: 166.61,123.17 166.55,123.2
S$12762
  Bottom 0: 166.55,123.2 166.49,123.23
S$12763
  Bottom 0: 166.49,123.23 166.43,123.25
S$12764
  Bottom 0: 166.43,123.25 166.35,123.25
S$12765
  Bottom 0: 166.35,123.25 165.09,123.25
S$12766
  Bottom 0: 165.09,123.25 165.02,123.25
S$12767
  Bottom 0: 165.02,123.25 164.96,123.23
S$12768
  Bottom 0: 164.96,123.23 164.89,123.2
S$12769
  Bottom 0: 164.89,123.2 164.84,123.17
S$12770
  Bottom 0: 164.84,123.17 164.78,123.12
S$12771
  Bottom 0: 164.78,123.12 164.22,122.56
S$12772
  Bottom 0: 164.22,122.56 164.22,122.58
S$12773
  Bottom 0: 164.22,122.58 164.16,122.63
S$12774
  Bottom 0: 164.16,122.63 164.09,122.67
S$12775
  Bottom 0: 164.09,122.67 164.02,122.68
S$12776
  Bottom 0: 164.02,122.68 163.57,122.68
S$12777
  Bottom 0: 163.57,122.68 163.57,122.81
S$12778
  Bottom 0: 163.57,122.81 163.51,123.03
S$12779
  Bottom 0: 163.51,123.03 163.35,123.19
S$12780
  Bottom 0: 163.35,123.19 163.13,123.25
S$12781
  Bottom 0: 163.13,123.25 162.78,123.25
S$12782
  Bottom 0: 162.78,123.25 161.7,124.33
S$12783
  Bottom 0: 161.7,124.33 161.76,124.47
S$12784
  Bottom 0: 161.76,124.47 161.8,124.79
S$12785
  Bottom 0: 161.8,124.79 161.76,125.11
S$12786
  Bottom 0: 161.76,125.11 161.63,125.41
S$12787
  Bottom 0: 161.63,125.41 161.42,125.66
S$12788
  Bottom 0: 161.42,125.66 161.16,125.85
S$12789
  Bottom 0: 161.16,125.85 160.85,125.96
S$12790
  Bottom 0: 160.85,125.96 160.53,125.98
S$12791
  Bottom 0: 160.53,125.98 160.21,125.91
S$12792
  Bottom 0: 160.21,125.91 159.92,125.77
S$12793
  Bottom 0: 159.92,125.77 159.68,125.54
S$12794
  Bottom 0: 159.68,125.54 159.51,125.27
S$12795
  Bottom 0: 159.51,125.27 159.43,124.95
S$12796
  Bottom 0: 159.43,124.95 159.43,124.63
S$12797
  Bottom 0: 159.43,124.63 159.51,124.31
S$12798
  Bottom 0: 159.51,124.31 159.68,124.04
S$12799
  Bottom 0: 159.68,124.04 159.92,123.81
S$12800
  Bottom 0: 159.92,123.81 160.21,123.67
S$12801
  Bottom 0: 160.21,123.67 160.53,123.6
S$12802
  Bottom 0: 160.53,123.6 160.85,123.62
S$12803
  Bottom 0: 160.85,123.62 161.07,123.7
S$12804
  Bottom 0: 161.07,123.7 162.12,122.65
S$12805
  Bottom 0: 162.12,122.65 162.09,122.63
S$12806
  Bottom 0: 162.09,122.63 162.04,122.58
S$12807
  Bottom 0: 162.04,122.58 162,122.5
S$12808
  Bottom 0: 162,122.5 161.99,122.43
S$12809
  Bottom 0: 161.99,122.43 161.99,120.65
S$12810
  Bottom 0: 161.99,120.65 162,120.58
S$12811
  Bottom 0: 162,120.58 155.9,120.58
S$12812
  Bottom 0: 155.9,120.58 155.86,120.8
S$12813
  Bottom 0: 155.86,120.8 155.73,121.08
S$12814
  Bottom 0: 155.73,121.08 155.52,121.3
S$12815
  Bottom 0: 155.52,121.3 155.26,121.45
S$12816
  Bottom 0: 155.26,121.45 154.97,121.51
S$12817
  Bottom 0: 154.97,121.51 154.66,121.49
S$12818
  Bottom 0: 154.66,121.49 154.38,121.38
S$12819
  Bottom 0: 154.38,121.38 154.14,121.19
S$12820
  Bottom 0: 154.14,121.19 153.97,120.94
S$12821
  Bottom 0: 153.97,120.94 153.88,120.66
S$12822
  Bottom 0: 153.88,120.66 153.88,120.35
S$12823
  Bottom 0: 153.88,120.35 153.97,120.06
S$12824
  Bottom 0: 153.97,120.06 154.14,119.81
S$12825
  Bottom 0: 154.14,119.81 154.38,119.62
S$12826
  Bottom 0: 154.38,119.62 154.66,119.51
S$12827
  Bottom 0: 154.66,119.51 154.97,119.49
S$12828
  Bottom 0: 154.97,119.49 155.26,119.56
S$12829
  Bottom 0: 155.26,119.56 155.5,119.69
S$12830
  Bottom 0: 155.5,119.69 164.13,119.69
S$12831
  Bottom 0: 164.13,119.69 164.21,119.7
S$12832
  Bottom 0: 164.21,119.7 164.27,119.72
S$12833
  Bottom 0: 164.27,119.72 164.33,119.74
S$12834
  Bottom 0: 164.33,119.74 164.39,119.78
S$12835
  Bottom 0: 164.39,119.78 164.45,119.82
S$12836
  Bottom 0: 164.45,119.82 164.7,120.08
S$12837
  Bottom 0: 164.7,120.08 164.74,120.13
S$12838
  Bottom 0: 164.74,120.13 164.78,120.19
S$12839
  Bottom 0: 164.78,120.19 164.81,120.25
S$12840
  Bottom 0: 164.81,120.25 164.82,120.32
S$12841
  Bottom 0: 164.82,120.32 164.83,120.39
S$12842
  Bottom 0: 164.83,120.39 164.83,120.78
S$12843
  Bottom 0: 164.83,120.78 164.92,120.67
S$12844
  Bottom 0: 164.92,120.67 165.2,120.5
S$12845
  Bottom 0: 165.2,120.5 165.51,120.41
S$12846
  Bottom 0: 165.51,120.41 165.83,120.41
S$12847
  Bottom 0: 165.83,120.41 165.96,120.45
S$12848
  Bottom 0: 165.96,120.45 169.41,117
S$12849
  Bottom 0: 169.41,117 169.41,114.62
S$12850
  Bottom 0: 169.41,114.62 169.22,114.87
S$12851
  Bottom 0: 169.22,114.87 168.96,115.1
S$12852
  Bottom 0: 168.96,115.1 168.64,115.25
S$12853
  Bottom 0: 168.64,115.25 168.29,115.31
S$12854
  Bottom 0: 168.29,115.31 167.94,115.29
S$12855
  Bottom 0: 167.94,115.29 167.62,115.18
S$12856
  Bottom 0: 167.62,115.18 167.32,115
S$12857
  Bottom 0: 167.32,115 167.08,114.74
S$12858
  Bottom 0: 167.08,114.74 166.91,114.43
S$12859
  Bottom 0: 166.91,114.43 166.82,114.09
S$12860
  Bottom 0: 166.82,114.09 166.82,113.75
S$12861
  Bottom 0: 166.82,113.75 166.91,113.41
S$12862
  Bottom 0: 166.91,113.41 166.96,113.3
S$12863
  Bottom 0: 166.96,113.3 163.85,110.19
S$12864
  Bottom 0: 163.85,110.19 162.6,110.19
S$12865
  Bottom 0: 162.6,110.19 162.6,110.2
S$12866
  Bottom 0: 162.6,110.2 162.88,110.42
S$12867
  Bottom 0: 162.88,110.42 163.08,110.71
S$12868
  Bottom 0: 163.08,110.71 163.21,111.03
S$12869
  Bottom 0: 163.21,111.03 163.26,111.38
S$12870
  Bottom 0: 163.26,111.38 163.21,111.72
S$12871
  Bottom 0: 163.21,111.72 163.08,112.05
S$12872
  Bottom 0: 163.08,112.05 162.88,112.33
S$12873
  Bottom 0: 162.88,112.33 162.6,112.56
S$12874
  Bottom 0: 162.6,112.56 162.29,112.71
S$12875
  Bottom 0: 162.29,112.71 161.94,112.77
S$12876
  Bottom 0: 161.94,112.77 161.59,112.75
S$12877
  Bottom 0: 161.59,112.75 161.26,112.64
S$12878
  Bottom 0: 161.26,112.64 161.24,112.63
S$12879
  Bottom 0: 161.24,112.63 160.67,113.2
S$12880
  Bottom 0: 160.67,113.2 160.61,113.24
S$12881
  Bottom 0: 160.61,113.24 160.55,113.28
S$12882
  Bottom 0: 160.55,113.28 160.49,113.3
S$12883
  Bottom 0: 160.49,113.3 160.43,113.32
S$12884
  Bottom 0: 160.43,113.32 160.35,113.33
S$12885
  Bottom 0: 160.35,113.33 155.79,113.33
S$12886
  Bottom 0: 155.79,113.33 155.73,113.46
S$12887
  Bottom 0: 155.73,113.46 155.52,113.67
S$12888
  Bottom 0: 155.52,113.67 155.26,113.83
S$12889
  Bottom 0: 155.26,113.83 154.97,113.89
S$12890
  Bottom 0: 154.97,113.89 154.66,113.87
S$12891
  Bottom 0: 154.66,113.87 154.38,113.76
S$12892
  Bottom 0: 154.38,113.76 154.14,113.57
S$12893
  Bottom 0: 154.14,113.57 153.97,113.33
S$12894
  Bottom 0: 153.97,113.33 153.88,113.03
S$12895
  Bottom 0: 153.88,113.03 153.88,112.73
S$12896
  Bottom 0: 153.88,112.73 153.97,112.44
S$12897
  Bottom 0: 153.97,112.44 154.14,112.19
S$12898
  Bottom 0: 154.14,112.19 154.38,112
S$12899
  Bottom 0: 154.38,112 154.66,111.89
S$12900
  Bottom 0: 154.66,111.89 154.97,111.87
S$12901
  Bottom 0: 154.97,111.87 155.26,111.94
S$12902
  Bottom 0: 155.26,111.94 155.52,112.09
S$12903
  Bottom 0: 155.52,112.09 155.73,112.31
S$12904
  Bottom 0: 155.73,112.31 155.79,112.44
S$12905
  Bottom 0: 155.79,112.44 160.17,112.44
S$12906
  Bottom 0: 160.17,112.44 160.61,111.99
S$12907
  Bottom 0: 160.61,111.99 160.56,111.89
S$12908
  Bottom 0: 160.56,111.89 160.47,111.55
S$12909
  Bottom 0: 160.47,111.55 160.47,111.21
S$12910
  Bottom 0: 160.47,111.21 160.56,110.87
S$12911
  Bottom 0: 160.56,110.87 160.73,110.56
S$12912
  Bottom 0: 160.73,110.56 160.97,110.3
S$12913
  Bottom 0: 160.97,110.3 161.14,110.19
S$12914
  Bottom 0: 161.14,110.19 147.97,110.19
S$12915
  Bottom 0: 164.4,114.17 164.85,114.22
S$12916
  Bottom 0: 164.85,114.22 165.27,114.35
S$12917
  Bottom 0: 165.27,114.35 165.67,114.56
S$12918
  Bottom 0: 165.67,114.56 166.01,114.84
S$12919
  Bottom 0: 166.01,114.84 166.3,115.19
S$12920
  Bottom 0: 166.3,115.19 166.51,115.58
S$12921
  Bottom 0: 166.51,115.58 166.64,116.01
S$12922
  Bottom 0: 166.64,116.01 166.69,116.46
S$12923
  Bottom 0: 166.69,116.46 166.64,116.91
S$12924
  Bottom 0: 166.64,116.91 166.51,117.33
S$12925
  Bottom 0: 166.51,117.33 166.3,117.73
S$12926
  Bottom 0: 166.3,117.73 166.01,118.07
S$12927
  Bottom 0: 166.01,118.07 165.67,118.36
S$12928
  Bottom 0: 165.67,118.36 165.27,118.57
S$12929
  Bottom 0: 165.27,118.57 164.85,118.7
S$12930
  Bottom 0: 164.85,118.7 164.4,118.75
S$12931
  Bottom 0: 164.4,118.75 163.95,118.7
S$12932
  Bottom 0: 163.95,118.7 163.52,118.57
S$12933
  Bottom 0: 163.52,118.57 163.13,118.36
S$12934
  Bottom 0: 163.13,118.36 162.78,118.07
S$12935
  Bottom 0: 162.78,118.07 162.5,117.73
S$12936
  Bottom 0: 162.5,117.73 162.28,117.33
S$12937
  Bottom 0: 162.28,117.33 162.16,116.91
S$12938
  Bottom 0: 162.16,116.91 162.11,116.46
S$12939
  Bottom 0: 162.11,116.46 162.16,116.01
S$12940
  Bottom 0: 162.16,116.01 162.28,115.58
S$12941
  Bottom 0: 162.28,115.58 162.5,115.19
S$12942
  Bottom 0: 162.5,115.19 162.78,114.84
S$12943
  Bottom 0: 162.78,114.84 163.13,114.56
S$12944
  Bottom 0: 163.13,114.56 163.52,114.35
S$12945
  Bottom 0: 163.52,114.35 163.95,114.22
S$12946
  Bottom 0: 163.95,114.22 164.4,114.17
S$12947
  Bottom 0: 296.57,111.17 296.6,111.36
S$12948
  Bottom 0: 296.6,111.36 296.55,111.7
S$12949
  Bottom 0: 296.55,111.7 296.42,112.03
S$12950
  Bottom 0: 296.42,112.03 296.21,112.31
S$12951
  Bottom 0: 296.21,112.31 295.95,112.54
S$12952
  Bottom 0: 295.95,112.54 295.63,112.69
S$12953
  Bottom 0: 295.63,112.69 295.29,112.75
S$12954
  Bottom 0: 295.29,112.75 294.94,112.73
S$12955
  Bottom 0: 294.94,112.73 294.83,112.69
S$12956
  Bottom 0: 294.83,112.69 294.52,112.75
S$12957
  Bottom 0: 294.52,112.75 294.17,112.73
S$12958
  Bottom 0: 294.17,112.73 293.84,112.62
S$12959
  Bottom 0: 293.84,112.62 293.55,112.44
S$12960
  Bottom 0: 293.55,112.44 293.31,112.18
S$12961
  Bottom 0: 293.31,112.18 293.14,111.87
S$12962
  Bottom 0: 293.14,111.87 293.12,111.8
S$12963
  Bottom 0: 293.12,111.8 289.95,111.8
S$12964
  Bottom 0: 289.95,111.8 289.2,112.55
S$12965
  Bottom 0: 289.2,112.55 289.22,112.58
S$12966
  Bottom 0: 289.22,112.58 289.26,112.88
S$12967
  Bottom 0: 289.26,112.88 289.22,113.18
S$12968
  Bottom 0: 289.22,113.18 289.09,113.46
S$12969
  Bottom 0: 289.09,113.46 288.88,113.67
S$12970
  Bottom 0: 288.88,113.67 288.62,113.83
S$12971
  Bottom 0: 288.62,113.83 288.33,113.89
S$12972
  Bottom 0: 288.33,113.89 288.02,113.87
S$12973
  Bottom 0: 288.02,113.87 287.74,113.76
S$12974
  Bottom 0: 287.74,113.76 287.54,113.6
S$12975
  Bottom 0: 287.54,113.6 287.54,119.78
S$12976
  Bottom 0: 287.54,119.78 287.74,119.62
S$12977
  Bottom 0: 287.74,119.62 288.02,119.51
S$12978
  Bottom 0: 288.02,119.51 288.33,119.49
S$12979
  Bottom 0: 288.33,119.49 288.62,119.56
S$12980
  Bottom 0: 288.62,119.56 288.88,119.71
S$12981
  Bottom 0: 288.88,119.71 289.09,119.93
S$12982
  Bottom 0: 289.09,119.93 289.22,120.2
S$12983
  Bottom 0: 289.22,120.2 289.26,120.5
S$12984
  Bottom 0: 289.26,120.5 289.22,120.8
S$12985
  Bottom 0: 289.22,120.8 289.09,121.08
S$12986
  Bottom 0: 289.09,121.08 288.88,121.3
S$12987
  Bottom 0: 288.88,121.3 288.62,121.45
S$12988
  Bottom 0: 288.62,121.45 288.33,121.51
S$12989
  Bottom 0: 288.33,121.51 288.02,121.49
S$12990
  Bottom 0: 288.02,121.49 287.74,121.38
S$12991
  Bottom 0: 287.74,121.38 287.54,121.22
S$12992
  Bottom 0: 287.54,121.22 287.54,122.42
S$12993
  Bottom 0: 287.54,122.42 294.56,122.42
S$12994
  Bottom 0: 294.56,122.42 294.56,120.64
S$12995
  Bottom 0: 294.56,120.64 294.57,120.56
S$12996
  Bottom 0: 294.57,120.56 294.62,120.49
S$12997
  Bottom 0: 294.62,120.49 294.67,120.44
S$12998
  Bottom 0: 294.67,120.44 294.74,120.4
S$12999
  Bottom 0: 294.74,120.4 294.82,120.39
S$13000
  Bottom 0: 294.82,120.39 297.23,120.39
S$13001
  Bottom 0: 297.23,120.39 297.3,120.4
S$13002
  Bottom 0: 297.3,120.4 297.37,120.44
S$13003
  Bottom 0: 297.37,120.44 297.43,120.49
S$13004
  Bottom 0: 297.43,120.49 297.47,120.56
S$13005
  Bottom 0: 297.47,120.56 297.48,120.64
S$13006
  Bottom 0: 297.48,120.64 297.48,120.86
S$13007
  Bottom 0: 297.48,120.86 297.5,120.83
S$13008
  Bottom 0: 297.5,120.83 297.74,120.64
S$13009
  Bottom 0: 297.74,120.64 298.02,120.53
S$13010
  Bottom 0: 298.02,120.53 298.32,120.51
S$13011
  Bottom 0: 298.32,120.51 298.44,120.53
S$13012
  Bottom 0: 298.44,120.53 298.53,120.48
S$13013
  Bottom 0: 298.53,120.48 298.85,120.39
S$13014
  Bottom 0: 298.85,120.39 299.17,120.39
S$13015
  Bottom 0: 299.17,120.39 299.48,120.48
S$13016
  Bottom 0: 299.48,120.48 299.76,120.66
S$13017
  Bottom 0: 299.76,120.66 299.85,120.77
S$13018
  Bottom 0: 299.85,120.77 299.85,117.31
S$13019
  Bottom 0: 299.85,117.31 299.85,117.32
S$13020
  Bottom 0: 299.85,117.32 299.63,117.72
S$13021
  Bottom 0: 299.63,117.72 299.35,118.06
S$13022
  Bottom 0: 299.35,118.06 299,118.35
S$13023
  Bottom 0: 299,118.35 298.61,118.56
S$13024
  Bottom 0: 298.61,118.56 298.18,118.69
S$13025
  Bottom 0: 298.18,118.69 297.73,118.73
S$13026
  Bottom 0: 297.73,118.73 297.35,118.69
S$13027
  Bottom 0: 297.35,118.69 296.97,118.73
S$13028
  Bottom 0: 296.97,118.73 296.52,118.69
S$13029
  Bottom 0: 296.52,118.69 296.1,118.56
S$13030
  Bottom 0: 296.1,118.56 295.7,118.35
S$13031
  Bottom 0: 295.7,118.35 295.36,118.06
S$13032
  Bottom 0: 295.36,118.06 295.07,117.72
S$13033
  Bottom 0: 295.07,117.72 294.86,117.32
S$13034
  Bottom 0: 294.86,117.32 294.73,116.9
S$13035
  Bottom 0: 294.73,116.9 294.69,116.45
S$13036
  Bottom 0: 294.69,116.45 294.73,116
S$13037
  Bottom 0: 294.73,116 294.86,115.58
S$13038
  Bottom 0: 294.86,115.58 295.07,115.18
S$13039
  Bottom 0: 295.07,115.18 295.36,114.83
S$13040
  Bottom 0: 295.36,114.83 295.7,114.55
S$13041
  Bottom 0: 295.7,114.55 296.1,114.34
S$13042
  Bottom 0: 296.1,114.34 296.52,114.21
S$13043
  Bottom 0: 296.52,114.21 296.97,114.16
S$13044
  Bottom 0: 296.97,114.16 297.35,114.2
S$13045
  Bottom 0: 297.35,114.2 297.73,114.16
S$13046
  Bottom 0: 297.73,114.16 298.18,114.21
S$13047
